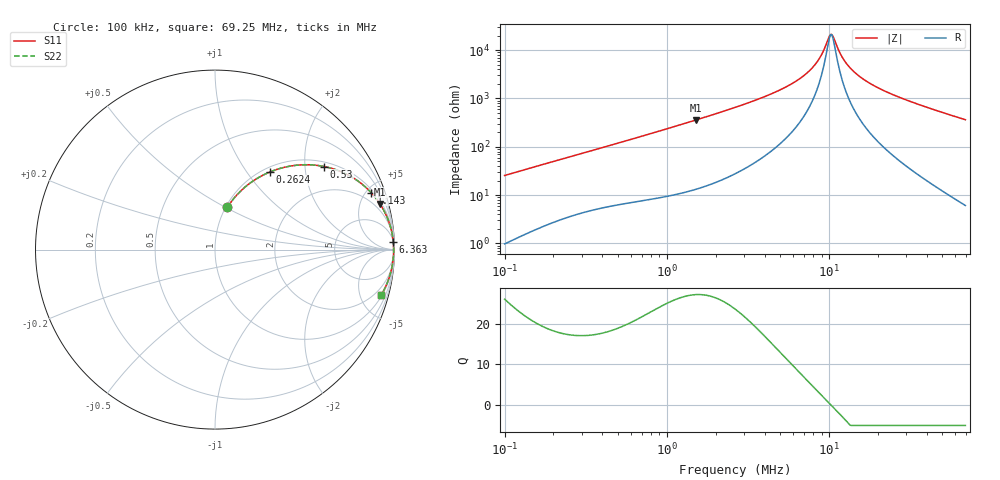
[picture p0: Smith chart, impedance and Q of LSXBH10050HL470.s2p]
! LSXBH10050HL470  S-PARAMETER MODEL  ( General Type )
! Model Generated by TAIYO YUDEN Corporation (http://www.ty-top.com)
! Version 3.0
! TAIYO YUDEN Control No. 180118NI43SB-FBB
! Copyright(c) 2007 TAIYO YUDEN CO.,LTD. All Rights Reserved.
! Product Description (link to TY-COMPAS)
! https://ds.yuden.co.jp/TYCOMPAS/or/detail?pn=LSXBH10050HL470M&u=M
! Products Name : Inductors
! Characteristics :
!  Inductance : 47 uH , SRF(min) : 7 MHz , DC Resistance(max) : 0.1196 Ohm
!  Rated Current : Saturation :2000 mA , Temp Rise : 1800 mA (40 degC)
!  Case Size : 10.0 x 9.8 / 0.394 x 0.386 [mm/inch] , Thickness : 5 / 0.197 [mm/inch]
!  (Conditions: Temperature = 25 degC , DC Bias Current/Voltage = 0A / 0V)
! External Node Assignments :
!  1  o---GGG---o  2
! GND o---------o GND
! Frequency Range : 0.1MHz  -  69.245953MHz  [ 402 STEP ]
# MHz S RI R 50
! Freq[MHz].  S11 Real  S11 Imag  S21 Real  S21 Imag  S12 Real  S12 Imag  S22 Real  S22 Imag
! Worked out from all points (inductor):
!   401 points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, 100 kHz to 69.25 MHz, reference 50 ohm
!   read as one part in series: L = 40.3 uH near 103.3 kHz
!   highest Q = 27.1 at 1.509 MHz (marker M1), where L = 37.8 uH
!   self-resonance near 10.22 MHz
!   S11 on the Smith chart (normalised r, x): 100 kHz: 1.02, +0.51; 262.4 kHz: 1.07, +1.29; 530 kHz: 1.13, +2.52; 1.143 MHz: 1.21, +5.39; 6.363 MHz: 6, +47; 69.25 MHz: 1.12, -7.26
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0.1  0.069 0.235  0.931 -0.235  0.931 -0.235  0.069 0.235
0.163316  0.1564 0.3388  0.8436 -0.3388  0.8436 -0.3388  0.1564 0.3388
0.262397  0.3041 0.4318  0.6959 -0.4318  0.6959 -0.4318  0.3041 0.4318
0.299065  0.3557 0.4503  0.6443 -0.4503  0.6443 -0.4503  0.3557 0.4503
0.53003  0.6085 0.4629  0.3915 -0.4629  0.3915 -0.4629  0.6085 0.4629
0.894401  0.8064 0.3748  0.1936 -0.3748  0.1936 -0.3748  0.8064 0.3748
1.143002  0.8699 0.3178  0.1301 -0.3178  0.1301 -0.3178  0.8699 0.3178
1.509259  0.9198 0.2538  0.0802 -0.2538  0.0802 -0.2538  0.9198 0.2538
2.631463  0.9711 0.1478  0.0289 -0.1478  0.0289 -0.1478  0.9711 0.1478
4.440468  0.9887 0.0778  0.0113 -0.0778  0.0113 -0.0778  0.9887 0.0778
6.362832  0.9934 0.0415  0.0066 -0.0415  0.0066 -0.0415  0.9934 0.0415
7.869792  0.9947 0.0226  0.00527 -0.0226  0.00527 -0.0226  0.9947 0.0226
8.824095  0.9951 0.0129  0.00488 -0.0129  0.00488 -0.0129  0.9951 0.0129
10.05722  0.9953 0.00202  0.00467 -0.00202  0.00467 -0.00202  0.9953 0.00202
10.39154  0.9953 -0.000693  0.00466 0.000693  0.00466 0.000693  0.9953 -0.000693
10.73698  0.9953 -0.00341  0.00467 0.00341  0.00467 0.00341  0.9953 -0.00341
12.23742  0.9952 -0.0143  0.00483 0.0143  0.00483 0.0143  0.9952 -0.0143
13.94754  0.9947 -0.0255  0.00526 0.0255  0.00526 0.0255  0.9947 -0.0255
17.25085  0.9934 -0.0446  0.00659 0.0446  0.00659 0.0446  0.9934 -0.0446
23.53582  0.9896 -0.0762  0.0104 0.0762  0.0104 0.0762  0.9896 -0.0762
37.81446  0.9759 -0.1382  0.0241 0.1382  0.0241 0.1382  0.9759 -0.1382
69.24595  0.9259 -0.2537  0.0741 0.2537  0.0741 0.2537  0.9259 -0.2537
